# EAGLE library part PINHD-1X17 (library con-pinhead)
PIN HEADER
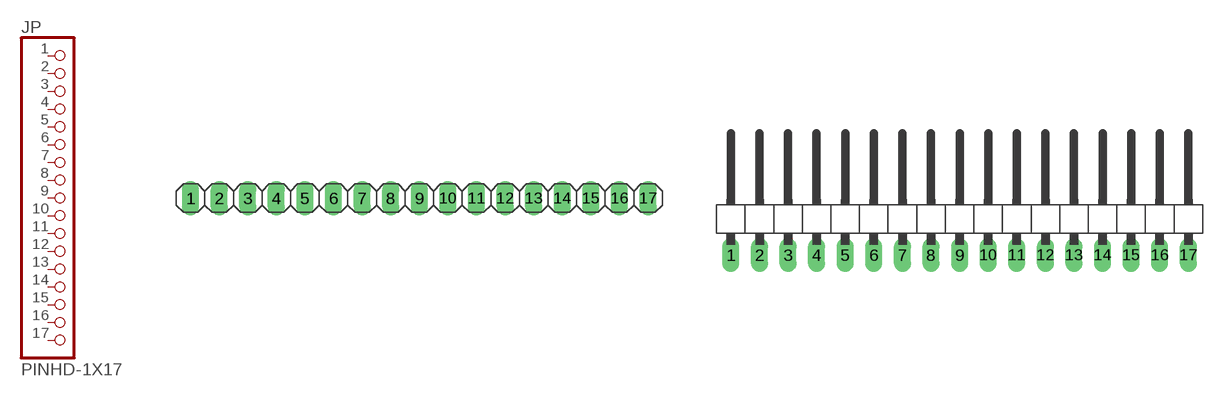
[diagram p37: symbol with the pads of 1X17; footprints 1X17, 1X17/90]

Designator prefix JP

## PINHD-1X17_2.54  [1X17]
1  1  pas
2  2  pas
3  3  pas
4  4  pas
5  5  pas
6  6  pas
7  7  pas
8  8  pas
9  9  pas
10  10  pas
11  11  pas
12  12  pas
13  13  pas
14  14  pas
15  15  pas
16  16  pas
17  17  pas

## PINHD-1X17_2.54-90°  [1X17/90]
Pads as for 1X17

## PINHD-1X17_2.00  [1X17M]
Pads as for 1X17

## PINHD-1X17_2.54-SMD  [1X17SMD]
Pads as for 1X17

## PINHD-1X17_2.54-SMD-90°  [1X17SMD/90]
Pads as for 1X17

## Footprint 1X17 (pad centres in mm)
PIN HEADER - 2.54
drill 1.016 long: 1 -20.32,0; 2 -17.78,0; 3 -15.24,0; 4 -12.7,0; 5 -10.16,0; 6 -7.62,0; 7 -5.08,0; 8 -2.54,0; 9 0,0; 10 2.54,0; 11 5.08,0; 12 7.62,0; 13 10.16,0; 14 12.7,0; 15 15.24,0; 16 17.78,0; 17 20.32,0

## Footprint 1X17/90 (pad centres in mm)
PIN HEADER - 2.54 90°
drill 1.016 long: 1 -20.32,-3.81; 2 -17.78,-3.81; 3 -15.24,-3.81; 4 -12.7,-3.81; 5 -10.16,-3.81; 6 -7.62,-3.81; 7 -5.08,-3.81; 8 -2.54,-3.81; 9 0,-3.81; 10 2.54,-3.81; 11 5.08,-3.81; 12 7.62,-3.81; 13 10.16,-3.81; 14 12.7,-3.81; 15 15.24,-3.81; 16 17.78,-3.81; 17 20.32,-3.81

## Footprint 1X17M (pad centres in mm)
PIN HEADER - 2
drill 0.914 square: 1 -16,0
drill 0.914: 2 -14,0; 3 -12,0; 4 -10,0; 5 -8,0; 6 -6,0; 7 -4,0; 8 -2,0; 9 0,0; 10 2,0; 11 4,0; 12 6,0; 13 8,0; 14 10,0; 15 12,0; 16 14,0; 17 16,0

## Footprint 1X17SMD (pad centres in mm)
PIN HEADER - 2.54 SMD
smd 1.016 x 3.302: 1 -1.27,1.27; 2 1.27,-1.27; 3 3.81,1.27; 4 6.35,-1.27; 5 8.89,1.27; 6 11.43,-1.27; 7 13.97,1.27; 8 16.51,-1.27; 9 19.05,1.27; 10 21.59,-1.27; 11 24.13,1.27; 12 26.67,-1.27; 13 29.21,1.27; 14 31.75,-1.27; 15 34.29,1.27; 16 36.83,-1.27; 17 39.37,1.27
